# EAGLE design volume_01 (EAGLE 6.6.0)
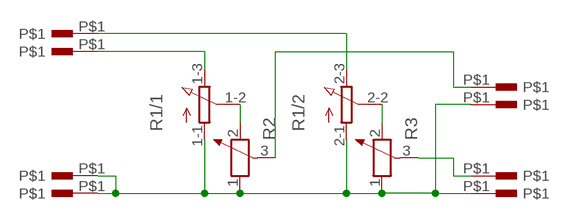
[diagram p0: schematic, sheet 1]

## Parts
R1  3RP/1610G  [3RP/1610G]
R2  POTENTIOMETER_PT-10  [PT-10]
R3  POTENTIOMETER_PT-10  [PT-10]
U$14  PIN  [PIN]
U$15  PIN  [PIN]
U$16  PIN  [PIN]
U$17  PIN  [PIN]
U$18  PIN  [PIN]
U$19  PIN  [PIN]
U$20  PIN  [PIN]
U$21  PIN  [PIN]

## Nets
GND: R1.1-1(/1:A) R1.2-1(/2:A) R2.1 R3.1 U$14.P$1 U$15.P$1 U$16.P$1 U$21.P$1
N$1: R1.1-2(/1:S) R2.2
N$3: R1.2-2(/2:S) R3.2
N$4: R3.3 U$20.P$1
N$5: R2.3 U$19.P$1
N$15: R1.1-3(/1:E) U$18.P$1
N$17: R1.2-3(/2:E) U$17.P$1

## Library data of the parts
R1 = pot:3RP/1610G: 16mm Potentiometer two level Source: http://www.alphapotentiometers.net/html/16mm_pot_2.html
R2 R3 = rcl:POTENTIOMETER_: Potentiometer
U$14-U$21 = lampy04:PIN

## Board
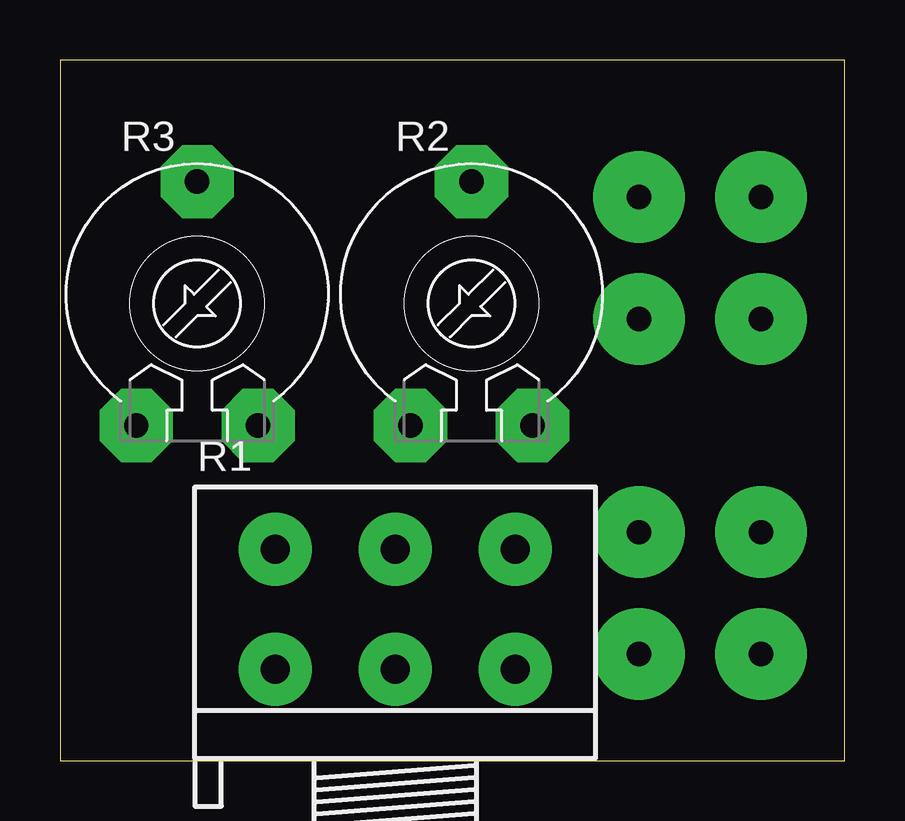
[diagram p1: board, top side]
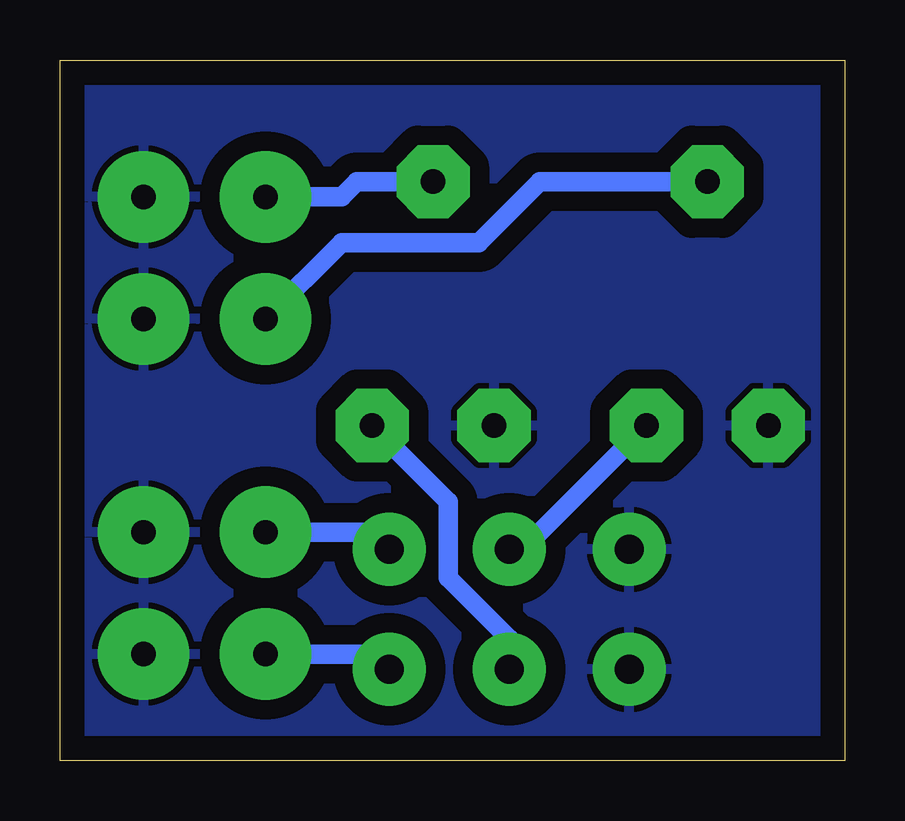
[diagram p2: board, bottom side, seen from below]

Size 32.69 x 29.2 mm. Coordinates in mm from the lower left corner, seen from the top.
Outline: 0,0 32.69,0 32.69,29.2 0,29.2 0,0
Copper layers (1*16): Top 0.035mm / dielectric 1.5mm / Bottom 0.035mm
Design rules "default": minimum track width 10mil, minimum drill 24mil, track to track 8mil, track to pad 8mil, pad to pad 8mil, via to via 8mil, smd to smd 8mil, copper to edge 40mil, drill to drill 8mil, minimum pad ring 10mil, minimum via ring 8mil, stop-mask expansion 4mil, vias tented up to drill 0mil, thermal gap 10mil

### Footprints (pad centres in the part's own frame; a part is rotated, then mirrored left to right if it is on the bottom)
3RP/1610G = drill 1.2 pad 3.048: 1-1 -5,0; 1-2 0,0; 1-3 5,0; 2-1 -5,5; 2-2 0,5; 2-3 5,5
PT-10 = drill 1.016 pad 3.048 octagon: 1 -2.54,-5.08; 2 2.54,-5.08; 3 0,5.08
PIN = drill 1.016 pad 3.81: P$1 0,0

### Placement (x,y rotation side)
R1  13.97,3.81 0 top
R2  17.14,19.05 0 top
R3  5.71,19.05 0 top
U$14  29.21,18.41 0 top
U$15  29.21,4.45 0 top
U$16  29.21,9.53 0 top
U$17  24.13,9.53 0 top
U$18  24.13,4.45 0 top
U$19  24.13,23.5 0 top
U$20  24.13,18.41 0 top
U$21  29.21,23.5 0 top

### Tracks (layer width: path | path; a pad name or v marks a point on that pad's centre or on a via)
GND
  pour Bottom (isolate 0.813): 0,0 33.02,0 33.02,29.21 0,29.21
N$1
  Bottom 0.813: R1.1-2 13.97,5.08 16.51,7.62 16.51,10.79 R2.2
N$3
  Bottom 0.813: R1.2-2 13.41,8.81 R3.2
N$4
  Bottom 0.813: R3.3 12.7,24.13 15.24,21.59 20.95,21.59 U$20.P$1
N$5
  Bottom 0.813: R2.3 20.32,24.13 20.95,23.5 U$19.P$1
N$15
  Bottom 0.813: R1.1-3 19.68,4.45 U$18.P$1
N$17
  Bottom 0.813: R1.2-3 19.68,9.53 U$17.P$1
